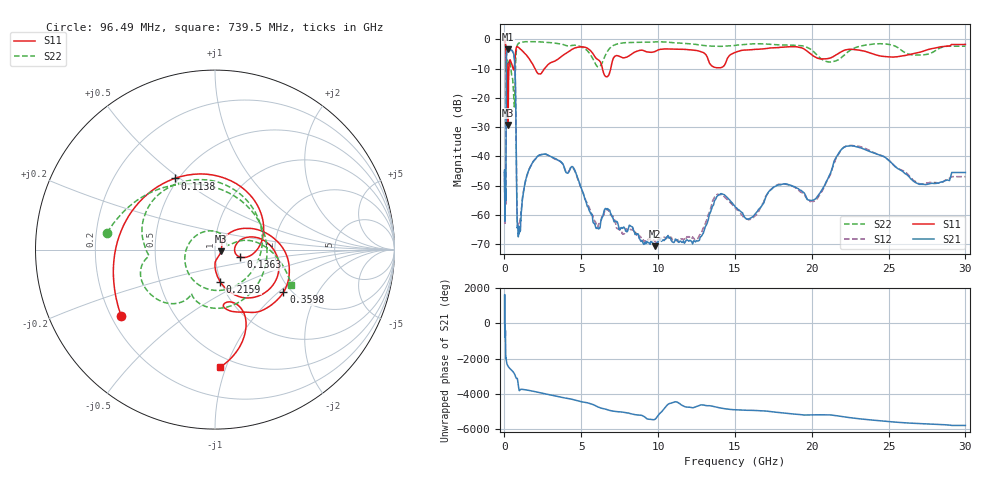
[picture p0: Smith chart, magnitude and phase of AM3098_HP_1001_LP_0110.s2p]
! Date/Time: Thu, Feb 28, 2019 8:41 AM
! Network Analyzer: Agilent Technologies E8364B Rev: A.07.50.67
! Sweep from 0.010 to 30.000 GHz, 1601 Points, Sweep Type: LOG
! Power Supply: 5.022 V, 0.002 A
# Hz S DB R 50
!freq MagS11 AngS11 MagS21 AngS21 MagS12 AngS12 MagS22 AngS22
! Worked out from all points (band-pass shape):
!   1601 points, 10 MHz to 30 GHz, reference 50 ohm
!   highest |S21| = -3.41 dB at 238.7 MHz (marker M1); lowest = -70.7 dB at 9.78 GHz (marker M2)
!   |S21| within 3 dB of the highest: 129.3 MHz to 644.3 MHz (515 MHz wide, 133 % of centre)
!   lowest |S11| = -29.2 dB at 237.5 MHz (marker M3), VSWR 1.07, Z = 53.4 - j1.08 ohm
!   |S11| at or under -10 dB: 199.1 MHz to 288.2 MHz (89.07 MHz wide, 36.6 % of centre); 1.993 GHz to 2.598 GHz (605.2 MHz wide, 26.4 % of centre); 6.379 GHz to 6.915 GHz (535.6 MHz wide, 8.06 % of centre)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
!   |S22| runs from -23.1 to -0.5 dB; largest |S21 - S12| = 0.011
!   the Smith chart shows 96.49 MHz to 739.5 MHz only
!   S11 on the Smith chart (normalised r, x): 96.49 MHz: 0.24, -0.30; 113.8 MHz: 0.48, +0.48; 136.3 MHz: 1.32, -0.11; 215.9 MHz: 0.99, -0.37; 359.8 MHz: 1.82, -1.08; 739.5 MHz: 0.42, -0.96
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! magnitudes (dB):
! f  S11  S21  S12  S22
! 10 MHz  -0.3  -45.5  -44.8  -0.5
! 38.04 MHz  -0.5  -58.3  -61.0  -0.8
! 96.49 MHz  -3.9  -44.6  -44.0  -4.3
! 113.8 MHz  -6.8  -17.4  -17.4  -10.6
! 136.3 MHz  -16.6  -5.2  -5.1  -11.0
! 144.7 MHz  -19.0  -4.5  -4.5  -10.6
! 215.9 MHz  -14.9  -3.6  -3.5  -8.2
! 237.5 MHz  -29.2  -3.4  -3.4  -8.6
! 238.7 MHz  -29.1  -3.4  -3.4  -8.6
! 359.8 MHz  -6.9  -3.8  -3.8  -7.7
! 550.5 MHz  -9.7  -4.3  -4.2  -14.6
! 646.1 MHz  -9.6  -6.5  -6.5  -23.0
! 739.5 MHz  -3.7  -24.2  -24.1  -6.6
! 821.5 MHz  -2.4  -59.9  -59.9  -2.2
! 903.4 MHz  -2.7  -67.4  -63.7  -1.4
! 2.084 GHz  -10.9  -40.4  -40.4  -0.8
! 4.458 GHz  -3.2  -43.6  -43.8  -2.0
! 7.926 GHz  -6.1  -65.6  -64.7  -1.1
! 9.78 GHz  -4.2  -70.7  -68.8  -0.8
! 20.1 GHz  -5.6  -54.9  -55.4  -4.1
! 22.67 GHz  -3.4  -36.4  -36.3  -3.2
! 30 GHz  -1.7  -45.5  -46.9  -2.3
